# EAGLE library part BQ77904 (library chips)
A battery protection chip with OV/UV/OT/UT
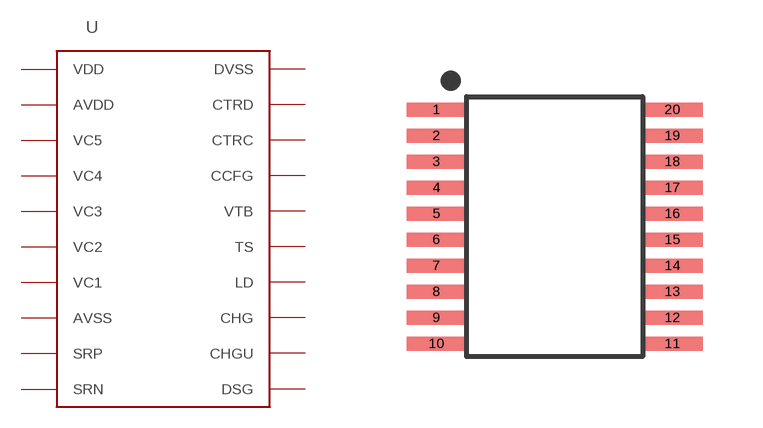
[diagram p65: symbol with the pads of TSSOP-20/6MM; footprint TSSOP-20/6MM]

Designator prefix U

## BQ77904 (DIGIKEY: 296-44599-5-ND; MANUFACTURER: TI; MOUSER: 595-BQ7790503PW; MPN: BQ7790503PW)  [TSSOP-20/6MM]
1  VDD
2  AVDD
3  VC5
4  VC4
5  VC3
6  VC2
7  VC1
8  AVSS
9  SRP
10  SRN
11  DSG
12  CHGU
13  CHG
14  LD
15  TS
16  VTB
17  CCFG
18  CTRC
19  CTRD
20  DVSS

## Footprint TSSOP-20/6MM (pad centres in mm)
smd 1.5 x 0.35: 1 -2.95,2.925; 2 -2.95,2.275; 3 -2.95,1.625; 4 -2.95,0.975; 5 -2.95,0.325; 6 -2.95,-0.325; 7 -2.95,-0.975; 8 -2.95,-1.625; 9 -2.95,-2.275; 10 -2.95,-2.925; 11 2.95,-2.925; 12 2.95,-2.275; 13 2.95,-1.625; 14 2.95,-0.975; 15 2.95,-0.325; 16 2.95,0.325; 17 2.95,0.975; 18 2.95,1.625; 19 2.95,2.275; 20 2.95,2.925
